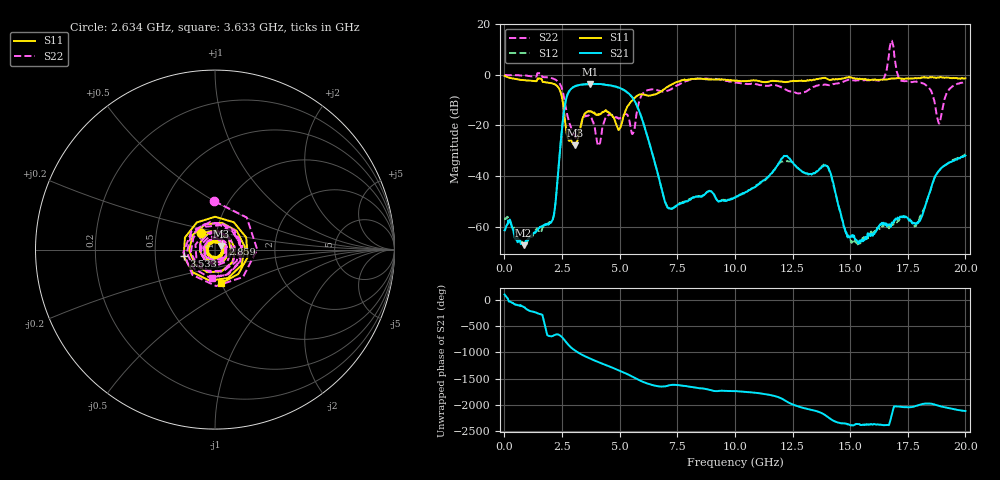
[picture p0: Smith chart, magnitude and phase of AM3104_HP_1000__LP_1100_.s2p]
!Created with skrf (http://scikit-rf.org).
# Hz S RI R 50.0
!freq ReS11 ImS11 ReS21 ImS21 ReS12 ImS12 ReS22 ImS22
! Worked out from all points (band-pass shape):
!   1601 points, 10 MHz to 20 GHz, reference 50 ohm
!   highest |S21| = -3.56 dB at 3.708 GHz (marker M1); lowest = -67.5 dB at 834.6 MHz (marker M2)
!   |S21| within 3 dB of the highest: 2.801 GHz to 5.283 GHz (2.482 GHz wide, 61.4 % of centre)
!   lowest |S11| = -27.9 dB at 3.083 GHz (marker M3), VSWR 1.08, Z = 53.6 + j2.13 ohm
!   |S11| at or under -10 dB: 2.521 GHz to 5.561 GHz (3.04 GHz wide, 75.2 % of centre)
!   |S22| runs from -28.1 to 13.6 dB; largest |S21 - S12| = 0.058
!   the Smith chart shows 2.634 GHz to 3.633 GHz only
!   S11 on the Smith chart (normalised r, x): 2.634 GHz: 0.84, +0.16; 2.859 GHz: 1.08, +0.07; 3.533 GHz: 0.70, -0.05; 3.633 GHz: 1.00, -0.39
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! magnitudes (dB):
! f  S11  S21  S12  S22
! 10 MHz  -0.4  -61.5  -57.0  0.0
! 834.6 MHz  -2.1  -67.5  -67.5  -0.2
! 2.096 GHz  -3.4  -57.3  -57.3  -1.4
! 2.634 GHz  -18.5  -11.6  -11.6  -11.4
! 2.859 GHz  -25.8  -5.9  -5.9  -19.9
! 3.083 GHz  -27.9  -4.4  -4.4  -24.8
! 3.346 GHz  -19.0  -3.8  -3.9  -19.1
! 3.533 GHz  -15.0  -3.7  -3.8  -16.0
! 3.633 GHz  -14.4  -3.7  -3.8  -16.1
! 3.708 GHz  -14.5  -3.6  -3.6  -16.8
! 5.545 GHz  -10.2  -8.8  -8.8  -23.4
! 6.682 GHz  -7.2  -40.1  -40.1  -6.2
! 7.169 GHz  -4.2  -52.8  -53.1  -5.9
! 10.01 GHz  -2.4  -48.6  -48.5  -3.1
! 12.17 GHz  -2.8  -32.1  -34.1  -5.6
! 13.34 GHz  -2.1  -39.3  -39.3  -5.2
! 14.02 GHz  -1.7  -36.3  -36.1  -4.0
! 15.06 GHz  -1.1  -63.9  -66.5  -1.9
! 16.68 GHz  -1.6  -59.3  -60.3  7.3
! 17.96 GHz  -1.3  -58.2  -58.1  -2.8
! 18.85 GHz  -1.0  -37.9  -38.1  -19.2
! 20 GHz  -1.3  -31.9  -31.5  -2.7
